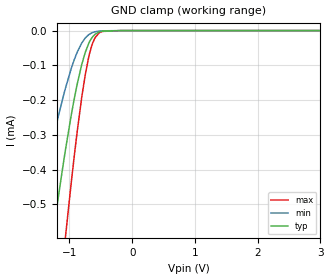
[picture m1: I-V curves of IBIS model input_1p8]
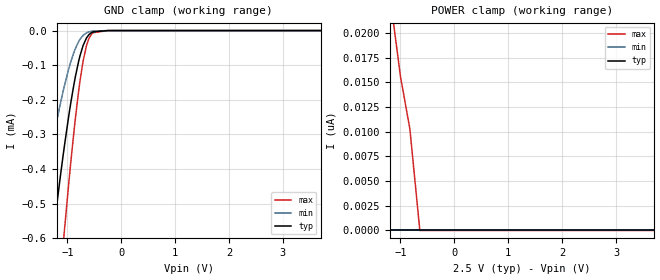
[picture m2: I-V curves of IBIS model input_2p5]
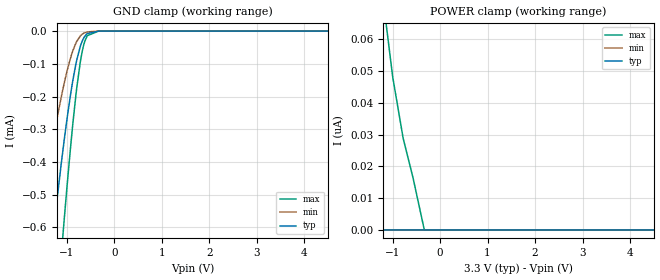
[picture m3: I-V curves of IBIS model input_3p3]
|Texas Instruments Incorporated
| Single Power Supply 2-INPUT POSITIVE OR GATE CMOS Logic Level Shifter
| Marketing part#   Digital Voltage Range   Package-type   #pins
| SN74LV1T32DBVR   1.6V - 5.5V   SOT-23   5
| SN74LV1T32DCKR   1.6V - 5.5V   SC70   5
[IBIS Ver]   4.1
[File name]   sn74lv1t32.ibs
[File Rev]   2.0
[Date]   12/19/2013
[Source]
| Texas Instruments Incorporated.
| Analog-eLab Design Center, HPA
| 12500 TI Blvd
| Dallas, TX -75243
[Notes]   Revision History:
| Rev 1.0: 11/08/2013
|  - Initial 5V model based on parent device SN74LVC1G32
| Rev 2.0: 12/19/2013
| - All New models across all voltage ranges.
| - Model generated from simulations in TISPICE
| - Model matched to SPICE simulation
| - C_comp although listed in numerical order of value are
|   obtained from varying PVT conditions. For PVT conditions for
|   each specific value refer the buffer description under
|   respective [Model]. IBIS model user is responsible for using
|   appropriate C_comp to simulate for Signal Integrity.
[Disclaimer]
| This model is designed as an aid for customers of Texas Instruments.
| TI and its licensors and suppliers make no warranties, either expressed
| or implied, with respect to this  model, including the warranties of
| merchantability or fitness for a particular purpose. The model is
| provided solely on an "as is" basis. The entire risk as to its quality
| and performance is with the customer.
[Copyright]
(C) Copyright 2013 Texas Instruments Incorporated.All rights reserved.
|   SN74LV1T32DBVR
[Component]   SN74LV1T32DBVR
[Manufacturer]   TI
[Package]   |5 SOT-23  -  DBV package
|   typ   min   max
R_pkg   0.06296   0.05007   0.07021
L_pkg   1.84798nH   1.48681nH   2.05223nH
C_pkg   0.26364pF   0.25321pF   0.27993pF
[Pin]  signal_name   model_name   R_pin   L_pin   C_pin
1   A   INPUT   0.07021   2.05223nH  0.27993pF
2   B   INPUT   0.05007   1.48681nH  0.25778pF
3   GND   GND   0.06861   2.45972nH  0.39618pF
4   Y   OUTPUT   0.06859   2.00489nH  0.25321pF
5   VCC   POWER   0.06799   1.99350nH  0.25274pF
|   SN74LV1T32DCKR
[Component]   SN74LV1T32DCKR
[Manufacturer]   TI
[Package]   |5 SC70   -  DCK package
|   typ   min   max
R_pkg   0.04798   0.04540   0.04946
L_pkg   1.59248nH   1.45465nH   1.69577nH
C_pkg   0.23694pF   0.23258pF   0.24105pF
[Pin]  signal_name   model_name   R_pin   L_pin   C_pin
1   A   INPUT   0.04907   1.62703nH  0.24105pF
2   B   INPUT   0.04540   1.45465nH  0.23719pF
3   GND   GND   0.04650   1.67316nH  0.26246pF
4   Y   OUTPUT   0.04946   1.69577nH  0.23258pF
5   VCC   POWER   0.04906   1.68894nH  0.23206pF
|   Model Selectors
[Model Selector] INPUT
input_1p8   1.8V  digital input
input_2p5   2.5V  digital input
input_3p3   3.3V  digital input
input_5p0   5.0V  digital input
[Model Selector] OUTPUT
output_1p8   1.8V  digital output
output_2p5   2.5V  digital output
output_3p3   3.3V  digital output
output_5p0   5.0V  digital output
| Models and submodels in the file (8): input_1p8 (Input), input_2p5 (Input), input_3p3 (Input), input_5p0 (Input), output_1p8 (Output), output_2p5 (Output), output_3p3 (Output), output_5p0 (Output)
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|   input_1p8 Model
[Model]   input_1p8
Model_type   Input
Vinl = 0.58
Vinh = 0.94
|   typ   min   max
|   (nom PVT)   (fast PVT)   (slow PVT)
C_comp   5.751e-13   5.699e-13   5.856e-13
[Model spec]
|subparameter
Vinl   0.58   0.58   0.58
Vinh   0.94   0.94   0.99
| Where nom  PVT is Nominal Process, 1.8V, 40C
|   Fast PVT is Strong Process,  1.98V, -40C
|   Slow PVT is Weak Process,   1.62V, 140C
[Voltage Range]   1.8   1.62   1.98
|Junction Temperature
[Temperature Range]   40   140   -40
[Power Clamp Reference]   1.8   1.62   1.98
[GND Clamp Reference]   0   0   0
[GND Clamp]
|   Voltage   I(typ)   I(min)   I(max)
-1.8V     -1.392mA   -816.3uA   -2.045mA
-1.547V   -994.8uA   -564.3uA   -1.522mA
-1.282V   -615.1uA   -328.7uA   -995.6uA
-1.194V   -500.9uA   -259.4uA   -830.2uA
-1.063V   -343.2uA   -165.8uA   -593.8uA
-926.8mV  -199.7uA   -85.67uA   -366.7uA
-806mV    -99.14uA   -36.43uA   -194.6uA
-748.6mV  -63.2uA    -21.49uA   -127.9uA
-676.8mV  -31.03uA   -9.897uA   -64.04uA
-589.9mV  -10.22uA   -3.38uA    -19.91uA
-473.4mV  -1.672uA   -717.2nA   -2.465uA
3.6V      0A         0A         0A
[POWER Clamp]
|   Voltage   I(typ)   I(min)   I(max)
-1.8V     0A         0A         0A
0V        0A         0A         0A
3.6V      0A         0A         0A
|   input_2p5 Model
[Model]   input_2p5
Model_type   Input
Vinl = 0.75
Vinh = 1.135
|   typ   min   max
|   (nom PVT)   (fast PVT)   (slow PVT)
C_comp   5.734e-13   5.699e-13   5.803e-13
[Model spec]
|subparameter
Vinl   0.75   0.75   0.75
Vinh   1.135   1.135   1.21
| Where nom  PVT is Nominal Process, 2.5V, 40C
|   Fast PVT is Strong Process,  2.75V, -40C
|   Slow PVT is Weak Process,   2.25V, 140C
[Voltage Range]   2.5   2.25   2.75
|Junction Temperature
[Temperature Range]   40   140   -40
[Power Clamp Reference]   2.5   2.25   2.75
[GND Clamp Reference]   0   0   0
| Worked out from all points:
|   GND clamp passes 1 mA (typ) near -1.55 V on its own axis
[GND Clamp]
|   Voltage   I(typ)   I(min)   I(max)
-2.5V     -2.611mA   -1.615mA   -3.557mA
-1.699V   -1.231mA   -713.1uA   -1.834mA
-1.543V   -989.5uA   -560.6uA   -1.513mA
-1.361V   -725.6uA   -396.3uA   -1.151mA
-1.22V    -535.2uA   -279.7uA   -879.2uA
-1.059V   -339.2uA   -163.2uA   -586.6uA
-934mV    -207.5uA   -89.51uA   -378.4uA
-790mV    -88.93uA   -31.82uA   -175.2uA
-642.5mV  -20.99uA   -6.604uA   -42.54uA
-520mV    -3.632uA   -1.353uA   -6.051uA
-250mV    -36.27nA   -32.15nA   -21.71nA
5V        0A         0A         0A
[POWER Clamp]
|   Voltage   I(typ)   I(min)   I(max)
-2.5V     0A         0A         215.1nA
-1.153V   0A         0A         22.01nA
-825.3mV  0A         0A         10.31nA
-640mV    0A         0A         0A
5V        0A         0A         0A
|   input_3p3 Model
[Model]   input_3p3
Model_type   Input
Vinl = 0.8
Vinh = 1.35
|   typ   min   max
|   (nom PVT)   (fast PVT)   (slow PVT)
C_comp   5.716e-13   5.682e-13   5.786e-13
[Model spec]
|subparameter
Vinl   0.8   0.8   0.8
Vinh   1.35   1.35   1.47
| Where nom  PVT is Nominal Process, 3.3V, 40C
|   Fast PVT is Strong Process,  3.6V, -40C
|   Slow PVT is Weak Process,   3V, 140C
[Voltage Range]   3.3   3   3.6
|Junction Temperature
[Temperature Range]   40   140   -40
[Power Clamp Reference]   3.3   3   3.6
[GND Clamp Reference]   0   0   0
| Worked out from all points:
|   GND clamp passes 1 mA (typ) near -1.55 V on its own axis
[GND Clamp]
|   Voltage   I(typ)   I(min)   I(max)
-3.3V     -4.135mA   -2.645mA   -5.346mA
-1.738V   -1.293mA   -752.7uA   -1.915mA
-1.538V   -982.8uA   -556.1uA   -1.503mA
-1.284V   -620.6uA   -331.4uA   -1.001mA
-1.11V    -399.6uA   -198.2uA   -677.4uA
-1.049V   -329.4uA   -157.2uA   -570.4uA
-866.4mV  -147.3uA   -58.45uA   -277uA
-712.8mV  -46.3uA    -14.97uA   -93.66uA
-620.4mV  -16.05uA   -5.051uA   -31.72uA
-567.6mV  -7.671uA   -2.562uA   -14.07uA
-330mV    -156.2nA   -100.4nA   -131.5nA
6.6V      0A         0A         0A
[POWER Clamp]
|   Voltage   I(typ)   I(min)   I(max)
-3.3V     19.36nA    0A         930.2nA
-3.041V   14.75nA    0A         755.5nA
-2.706V   10.21nA    0A         559.7nA
-2.62V    0A         0A         514.6nA
-1.198V   0A         0A         72.59nA
-996mV    0A         0A         48.13nA
-775.5mV  0A         0A         28.82nA
-567.6mV  0A         0A         16.38nA
-330mV    0A         0A         0A
6.6V      0A         0A         0A
